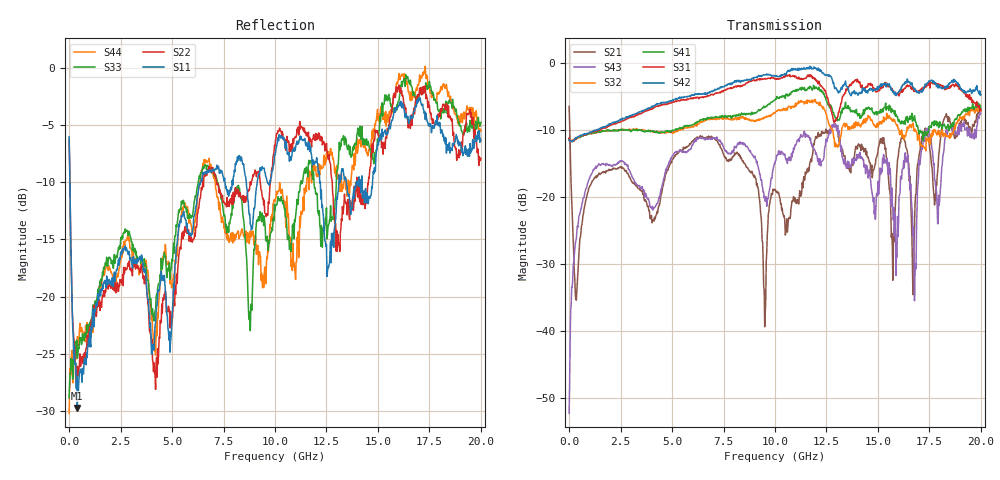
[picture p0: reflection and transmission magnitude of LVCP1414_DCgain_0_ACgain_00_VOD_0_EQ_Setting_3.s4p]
!Agilent Technologies,N5230A,MY46400459,A.07.50.48
!Agilent N5230A: A.07.50.48
!Date: Tuesday, April 17, 2012 18:34:22
!Correction: S11(Full 4 Port(1,2,3,4))
!S12(Full 4 Port(1,2,3,4))
!S13(Full 4 Port(1,2,3,4))
!S14(Full 4 Port(1,2,3,4))
!S21(Full 4 Port(1,2,3,4))
!S22(Full 4 Port(1,2,3,4))
!S23(Full 4 Port(1,2,3,4))
!S24(Full 4 Port(1,2,3,4))
!S31(Full 4 Port(1,2,3,4))
!S32(Full 4 Port(1,2,3,4))
!S33(Full 4 Port(1,2,3,4))
!S34(Full 4 Port(1,2,3,4))
!S41(Full 4 Port(1,2,3,4))
!S42(Full 4 Port(1,2,3,4))
!S43(Full 4 Port(1,2,3,4))
!S44(Full 4 Port(1,2,3,4))
!S4P File: Measurements: <S11,S12,S13,S14>,
!<S21,S22,S23,S24>,
!<S31,S32,S33,S34>,
!<S41,S42,S43,S44>:
# Hz S  dB  R 50
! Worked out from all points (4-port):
!   801 points, 300 kHz to 20 GHz, reference 50 ohm
!   strongest paths, dB at 300 kHz, 5 GHz, 10 GHz, 15 GHz, 20 GHz:
!     S42: -11.5, -5.6, -2.0, -3.6, -4.7
!     S31: -11.2, -5.9, -2.4, -4.2, -7.1
!     S41: -11.3, -10.1, -5.5, -7.4, -6.8
!     S32: -11.4, -10.4, -7.4, -9.6, -7.2
!     S43: -52.2, -13.9, -15.0, -17.6, -7.5
!     S21: -6.5, -14.5, -18.9, -13.2, -7.1
!   lowest |S11| = -29.7 dB at 400.3 MHz (marker M1), VSWR 1.07, Z = 53 + j1.46 ohm
!   |S11| at or under -10 dB: 37.6 MHz to 6.375 GHz (6.337 GHz wide, 198 % of centre); 8.606 GHz to 9.139 GHz (533.1 MHz wide, 6.01 % of centre); 12.2 GHz to 13.1 GHz (899.6 MHz wide, 7.11 % of centre)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
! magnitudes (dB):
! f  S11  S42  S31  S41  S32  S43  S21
! 300 kHz  -6.0  -11.5  -11.2  -11.3  -11.4  -52.2  -6.5
! 400.3 MHz  -29.7  -11.1  -11.1  -11.1  -11.2  -24.3  -32.3
! 6.325 GHz  -10.1  -4.7  -5.2  -8.7  -9.0  -11.2  -11.0
! 10.13 GHz  -6.3  -2.0  -2.4  -5.2  -7.1  -13.8  -19.4
! 12.73 GHz  -17.0  -2.1  -7.1  -6.6  -9.7  -9.9  -10.1
! 16.8 GHz  -3.5  -3.9  -4.0  -8.4  -9.9  -31.5  -21.1
! 20 GHz  -6.4  -4.7  -7.1  -6.8  -7.2  -7.5  -7.1
